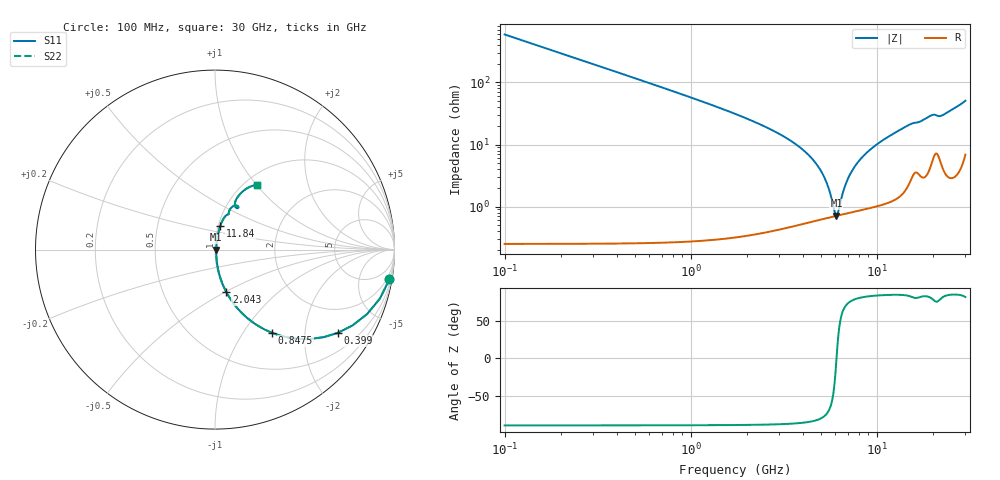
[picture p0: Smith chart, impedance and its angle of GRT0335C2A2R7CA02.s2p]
!Murata Part Number: GRT0335C2A2R7CA02
!These Parameters are Measured in Series Mode Connection
!Data Generated on Jun 19, 2026
!  o--ll--o
!Port1  Port2
!  o------o
!Operation Temp=25[degC], DC Bias Voltage=0[V]
!Freq. Start=100[MHz] Stop=30[GHz] 401[Steps]
# Hz S RI R 50
!Freq.(Hz) S11(Real) S11(Imag) S21(Real) S21(Imag) S12(Real) S12(Imag) S22(Real) S22(Imag)
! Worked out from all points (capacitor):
!   401 points, 100 MHz to 30 GHz, reference 50 ohm
!   read as one part in series: C = 2.7 pF near 249.5 MHz
!   lowest |Z| = 712 mohm at 6.08 GHz (marker M1)
!   series resonance near 6.086 GHz, so ESL is about 250 pH
!   S11 on the Smith chart (normalised r, x): 100 MHz: 1, -12; 399 MHz: 1.01, -2.94; 847.5 MHz: 1.01, -1.36; 2.043 GHz: 1.01, -0.51; 11.84 GHz: 1.02, +0.28; 30 GHz: 1.14, +1.00
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1e8  0.9719 -0.1649  0.0281 0.1649  0.0281 0.1649  0.9719 -0.1649
3.99e8  0.6836 -0.4642  0.3164 0.4642  0.3164 0.4642  0.6836 -0.4642
6.2325e8  0.4668 -0.4975  0.5332 0.4975  0.5332 0.4975  0.4668 -0.4975
8.475e8  0.3178 -0.4637  0.6822 0.4637  0.6822 0.4637  0.3178 -0.4637
1.296e9  0.1599 -0.3631  0.8401 0.3631  0.8401 0.3631  0.1599 -0.3631
2.0435e9  0.0639 -0.2379  0.9361 0.2379  0.9361 0.2379  0.0639 -0.2379
4.1365e9  0.011 -0.0746  0.989 0.0746  0.989 0.0746  0.011 -0.0746
5.10825e9  0.00735 -0.0332  0.9927 0.0332  0.9927 0.0332  0.00735 -0.0332
5.482e9  0.00696 -0.0197  0.993 0.0197  0.993 0.0197  0.00696 -0.0197
5.9305e9  0.00697 -0.00486  0.993 0.00486  0.993 0.00486  0.00697 -0.00486
6.08e9  0.00707 -0.000174  0.9929 0.000174  0.9929 0.000174  0.00707 -0.000174
6.2295e9  0.00721 0.0044  0.9928 -0.0044  0.9928 -0.0044  0.00721 0.0044
6.8275e9  0.00813 0.0217  0.9919 -0.0217  0.9919 -0.0217  0.00813 0.0217
7.50025e9  0.00973 0.0395  0.9903 -0.0395  0.9903 -0.0395  0.00973 0.0395
8.54675e9  0.0132 0.0647  0.9868 -0.0647  0.9868 -0.0647  0.0132 0.0647
1.01165e10  0.02 0.0988  0.98 -0.0988  0.98 -0.0988  0.02 0.0988
1.183575e10  0.03 0.1331  0.97 -0.1331  0.97 -0.1331  0.03 0.1331
1.505e10  0.0624 0.1905  0.9376 -0.1905  0.9376 -0.1905  0.0624 0.1905
2.005825e10  0.1224 0.245  0.8776 -0.245  0.8776 -0.245  0.1224 0.245
2.185225e10  0.1157 0.2349  0.8843 -0.2349  0.8843 -0.2349  0.1157 0.2349
2.50665e10  0.1306 0.2989  0.8694 -0.2989  0.8694 -0.2989  0.1306 0.2989
3e10  0.2331 0.3598  0.7669 -0.3598  0.7669 -0.3598  0.2331 0.3598
